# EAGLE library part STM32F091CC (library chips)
Description: STM32F091CC from STMicroelectronics, an ARM-based 32-bit MCU with 256 kB Flash, 32kB of SRAM and a Cortex M0
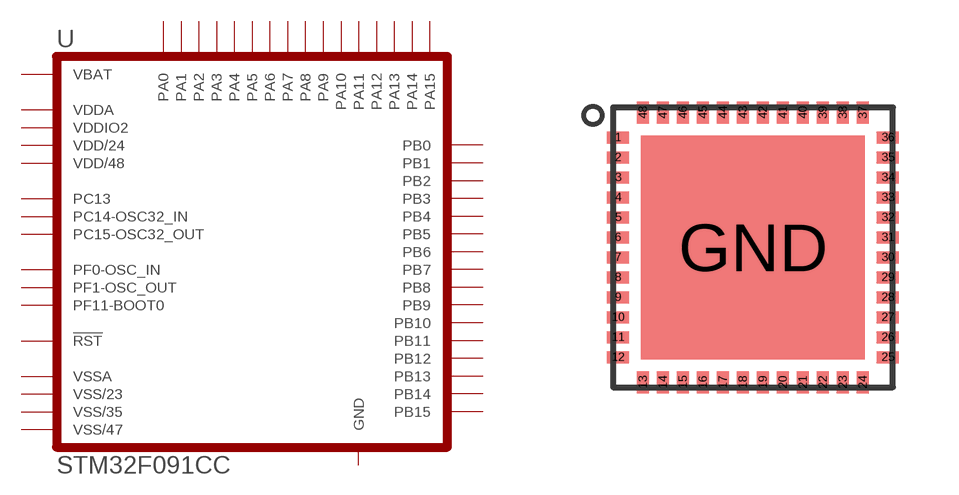
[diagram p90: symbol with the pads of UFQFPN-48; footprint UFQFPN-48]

Designator prefix U

## STM32F091CC (DATASHEET: https://www.st.com/resource/en/datasheet/stm32f091cc.pdf; DESCRIPTION: IC MCU 32BIT 256KB FLASH 48QFPN; DIGIKEY: 497-15813-ND; MANUFACTURER: STMicroelectronics; MOUSER: 511-STM32F091CCU6; MPN: STM32F091CCU6)  [UFQFPN-48]
1  VBAT  pwr
2  PC13
3  PC14-OSC32_IN
4  PC15-OSC32_OUT
5  PF0-OSC_IN
6  PF1-OSC_OUT
7  !RST
8  VSSA  pwr
9  VDDA  pwr
10  PA0
11  PA1
12  PA2
13  PA3
14  PA4
15  PA5
16  PA6
17  PA7
18  PB0
19  PB1
20  PB2
21  PB10
22  PB11
23  VSS/23  pwr
24  VDD/24  pwr
25  PB12
26  PB13
27  PB14
28  PB15
29  PA8
30  PA9
31  PA10
32  PA11
33  PA12
34  PA13
35  VSS/35  pwr
36  VDDIO2  pwr
37  PA14
38  PA15
39  PB3
40  PB4
41  PB5
42  PB6
43  PB7
44  PF11-BOOT0
45  PB8
46  PB9
47  VSS/47  pwr
48  VDD/48  pwr
GND  GND  pwr

## Footprint UFQFPN-48 (pad centres in mm)
Description: Footprint by STMicroelectronics for the STM32F091CC
smd 0.55 x 0.3: 1 -3.375,2.75; 2 -3.375,2.25; 3 -3.375,1.75; 4 -3.375,1.25; 5 -3.375,0.75; 6 -3.375,0.25; 7 -3.375,-0.25; 8 -3.375,-0.75; 9 -3.375,-1.25; 10 -3.375,-1.75; 11 -3.375,-2.25; 12 -3.375,-2.75; 25 3.375,-2.75; 26 3.375,-2.25; 27 3.375,-1.75; 28 3.375,-1.25; 29 3.375,-0.75; 30 3.375,-0.25; 31 3.375,0.25; 32 3.375,0.75; 33 3.375,1.25; 34 3.375,1.75; 35 3.375,2.25; 36 3.375,2.75
smd 0.3 x 0.55: 13 -2.75,-3.375; 14 -2.25,-3.375; 15 -1.75,-3.375; 16 -1.25,-3.375; 17 -0.75,-3.375; 18 -0.25,-3.375; 19 0.25,-3.375; 20 0.75,-3.375; 21 1.25,-3.375; 22 1.75,-3.375; 23 2.25,-3.375; 24 2.75,-3.375; 37 2.75,3.375; 38 2.25,3.375; 39 1.75,3.375; 40 1.25,3.375; 41 0.75,3.375; 42 0.25,3.375; 43 -0.25,3.375; 44 -0.75,3.375; 45 -1.25,3.375; 46 -1.75,3.375; 47 -2.25,3.375; 48 -2.75,3.375
smd 5.6 x 5.6: GND 0,0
